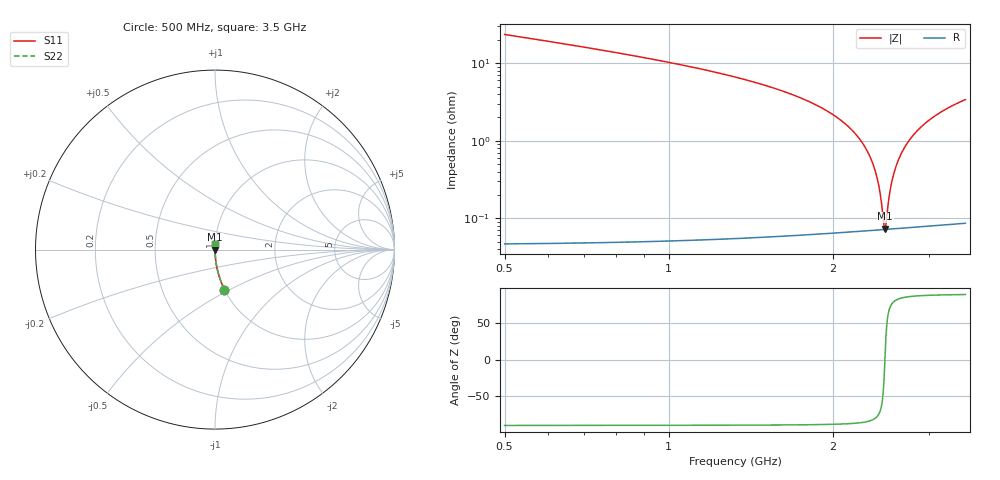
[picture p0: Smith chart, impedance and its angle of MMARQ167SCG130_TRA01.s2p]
! MMARQ167SCG130_TRA01  S-PARAMETER MODEL  ( General Type )
! Model Generated by TAIYO YUDEN Corporation (http://www.ty-top.com)
! Version 1.0
! TAIYO YUDEN Control No. 160201
! Copyright(c) 2016 TAIYO YUDEN CO.,LTD. All Rights Reserved.
! Product Description (link to TY-COMPAS)
! https://ds.yuden.co.jp/TYCOMPAS/or/detail?pn=MMARQ167SCG130JTRA01&u=M
! Products Name : Multilayer Ceramic Capacitors
! Characteristics :
!  Capacitance : 13 pF , Rated Voltage : 250V , TCC : CG / C0G
!  Case Size : 1.6 x 0.8 / 0.063 x 0.031 [mm/inch] , Thickness : 0.7 / 0.028 [mm/inch]
!  (Conditions: Temperature = 25 degC , DC Bias Current/Voltage = 0A / 0V)
! External Node Assignments :
!  1  o---| |---o  2
! GND o---------o GND
! Frequency Range : 500MHz  -  3500MHz  [ 401 STEP ]
# MHz S RI R 50
! Freq[MHz].  S11 Real  S11 Imag  S21 Real  S21 Imag  S12 Real  S12 Imag  S22 Real  S22 Imag
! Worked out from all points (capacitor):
!   401 points, 500 MHz to 3.5 GHz, reference 50 ohm
!   read as one part in series: C = 13 pF near 515 MHz
!   lowest |Z| = 73 mohm at 2.495 GHz (marker M1)
!   series resonance near 2.491 GHz, so ESL is about 310 pH
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500  0.0528 -0.2227  0.9472 0.2227  0.9472 0.2227  0.0528 -0.2227
1002.5  0.0109 -0.1012  0.9891 0.1012  0.9891 0.1012  0.0109 -0.1012
1505  0.00323 -0.0515  0.9968 0.0515  0.9968 0.0515  0.00323 -0.0515
1790  0.0017 -0.033  0.9983 0.033  0.9983 0.033  0.0017 -0.033
2000  0.00111 -0.0217  0.9989 0.0217  0.9989 0.0217  0.00111 -0.0217
2202.5  0.000818 -0.0121  0.9992 0.0121  0.9992 0.0121  0.000818 -0.0121
2337.5  0.000731 -0.00626  0.9993 0.00626  0.9993 0.00626  0.000731 -0.00626
2382.5  0.000718 -0.00438  0.9993 0.00438  0.9993 0.00438  0.000718 -0.00438
2412.5  0.000713 -0.00316  0.9993 0.00316  0.9993 0.00316  0.000713 -0.00316
2442.5  0.000712 -0.00194  0.9993 0.00194  0.9993 0.00194  0.000712 -0.00194
2480  0.000714 -0.000451  0.9993 0.000451  0.9993 0.000451  0.000714 -0.000451
2495  0.000716 0.00014  0.9993 -0.00014  0.9993 -0.00014  0.000716 0.00014
2502.5  0.000717 0.000435  0.9993 -0.000435  0.9993 -0.000435  0.000717 0.000435
2540  0.000726 0.00189  0.9993 -0.00189  0.9993 -0.00189  0.000726 0.00189
2562.5  0.000733 0.00276  0.9993 -0.00276  0.9993 -0.00276  0.000733 0.00276
2600  0.000749 0.00418  0.9993 -0.00418  0.9993 -0.00418  0.000749 0.00418
2652.5  0.000777 0.00614  0.9992 -0.00614  0.9992 -0.00614  0.000777 0.00614
2720  0.000824 0.00861  0.9992 -0.00861  0.9992 -0.00861  0.000824 0.00861
2795  0.000888 0.0113  0.9991 -0.0113  0.9991 -0.0113  0.000888 0.0113
3005  0.00113 0.0185  0.9989 -0.0185  0.9989 -0.0185  0.00113 0.0185
3230  0.00148 0.0257  0.9985 -0.0257  0.9985 -0.0257  0.00148 0.0257
3500  0.00201 0.0339  0.998 -0.0339  0.998 -0.0339  0.00201 0.0339
